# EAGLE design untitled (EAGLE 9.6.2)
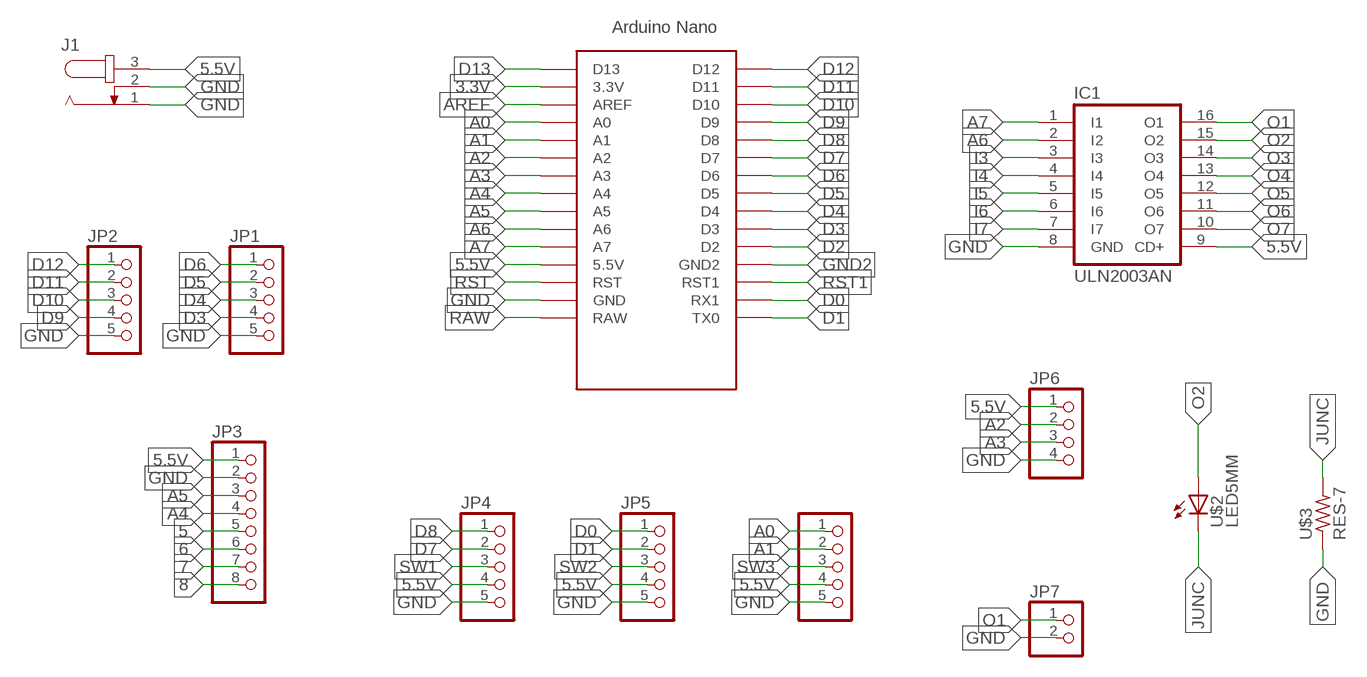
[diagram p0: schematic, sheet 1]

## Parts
3_ENCODERS  PINHD-1X5  [1X05]
IC1  ULN2003AN  [DIL16]
J1  JACK-PLUG0  [SPC4077]
JP1  PINHD-1X5  [1X05]
JP2  PINHD-1X5  [1X05]
JP3  PINHD-1X8  [1X08]
JP4  PINHD-1X5  [1X05]
JP5  PINHD-1X5  [1X05]
JP6  PINHD-1X4  [1X04]
JP7  PINHD-1X2  [1X02]
U$1  ARDUINO_NANO  [NANO]
U$2  LED5MM  [LED5MM]
U$3  RES-7  [0204/7]

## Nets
3.3V: U$1.3.3V
5: JP3.5
5.5V: 3_ENCODERS.4 IC1.9(CD+) J1.3 JP3.1 JP4.4 JP5.4 JP6.1 U$1.5V(5.5V)
6: JP3.6
7: JP3.7
8: JP3.8
A0: 3_ENCODERS.1 U$1.A0
A1: 3_ENCODERS.2 U$1.A1
A2: JP6.2 U$1.A2
A3: JP6.3 U$1.A3
A4: JP3.4 U$1.A4
A5: JP3.3 U$1.A5
A6: IC1.2(I2) U$1.A6
A7: IC1.1(I1) U$1.A7
AREF: U$1.AREF
D0: JP5.1 U$1.RX1
D1: JP5.2 U$1.TX0
D2: U$1.D2
D3: JP1.4 U$1.D3
D4: JP1.3 U$1.D4
D5: JP1.2 U$1.D5
D6: JP1.1 U$1.D6
D7: JP4.2 U$1.D7
D8: JP4.1 U$1.D8
D9: JP2.4 U$1.D9
D10: JP2.3 U$1.D10
D11: JP2.2 U$1.D11
D12: JP2.1 U$1.D12
D13: U$1.D13
GND: 3_ENCODERS.5 IC1.8(GND) J1.1 J1.2 JP1.5 JP2.5 JP3.2 JP4.5 JP5.5 JP6.4 JP7.2 U$1.GND U$3.1
GND2: U$1.GND1(GND2)
I3: IC1.3(I3)
I4: IC1.4(I4)
I5: IC1.5(I5)
I6: IC1.6(I6)
I7: IC1.7(I7)
JUNC: U$2.K(C) U$3.2
O1: IC1.16(O1) JP7.1
O2: IC1.15(O2) U$2.A
O3: IC1.14(O3)
O4: IC1.13(O4)
O5: IC1.12(O5)
O6: IC1.11(O6)
O7: IC1.10(O7)
RAW: U$1.RAW
RST: U$1.RST
RST1: U$1.RST1
SW1: JP4.3
SW2: JP5.3
SW3: 3_ENCODERS.3

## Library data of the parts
3_ENCODERS JP1 JP2 JP4 JP5 = MIA-Training:PINHD-1X5: PIN HEADER
IC1 = MIA-Training:ULN2003A: DRIVER ARRAY
J1 = con-jack:JACK-PLUG: DC POWER JACK Power Jack, DC, Right Angle, Through Hole, Rated 5A at 16VDC, PC Terminals Distributor: Farnell (www.Farnell.de) Drawing: 84N1161.pdf / 84N1162.pdf Manufacturer: SPC Technology (www.spctechnology.com) Type: SPC4077 / SPC 4078; OC_FARNELL: unknown; OC_NEWARK: unknown
JP3 = MIA-Training:PINHD-1X8: PIN HEADER
JP6 = MIA-Training:PINHD-1X4: PIN HEADER
JP7 = MIA-Training:PINHD-1X2: PIN HEADER
U$1 = MIA-Training:ARDUINO_NANO: Arduino Nano
U$2 = MIA-Training:LED5MM
U$3 = MIA-Training:RES-7

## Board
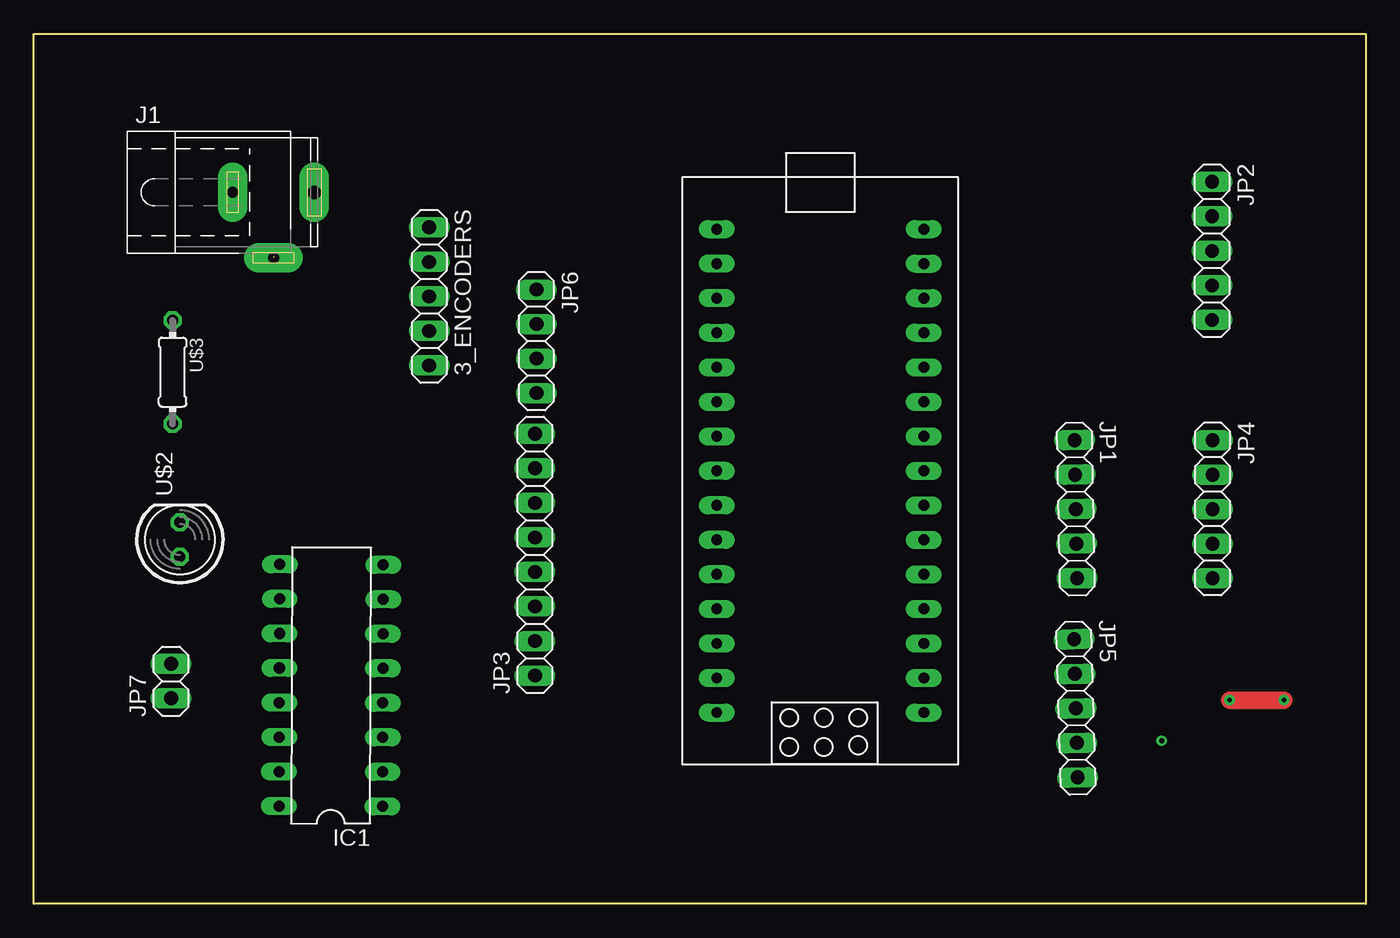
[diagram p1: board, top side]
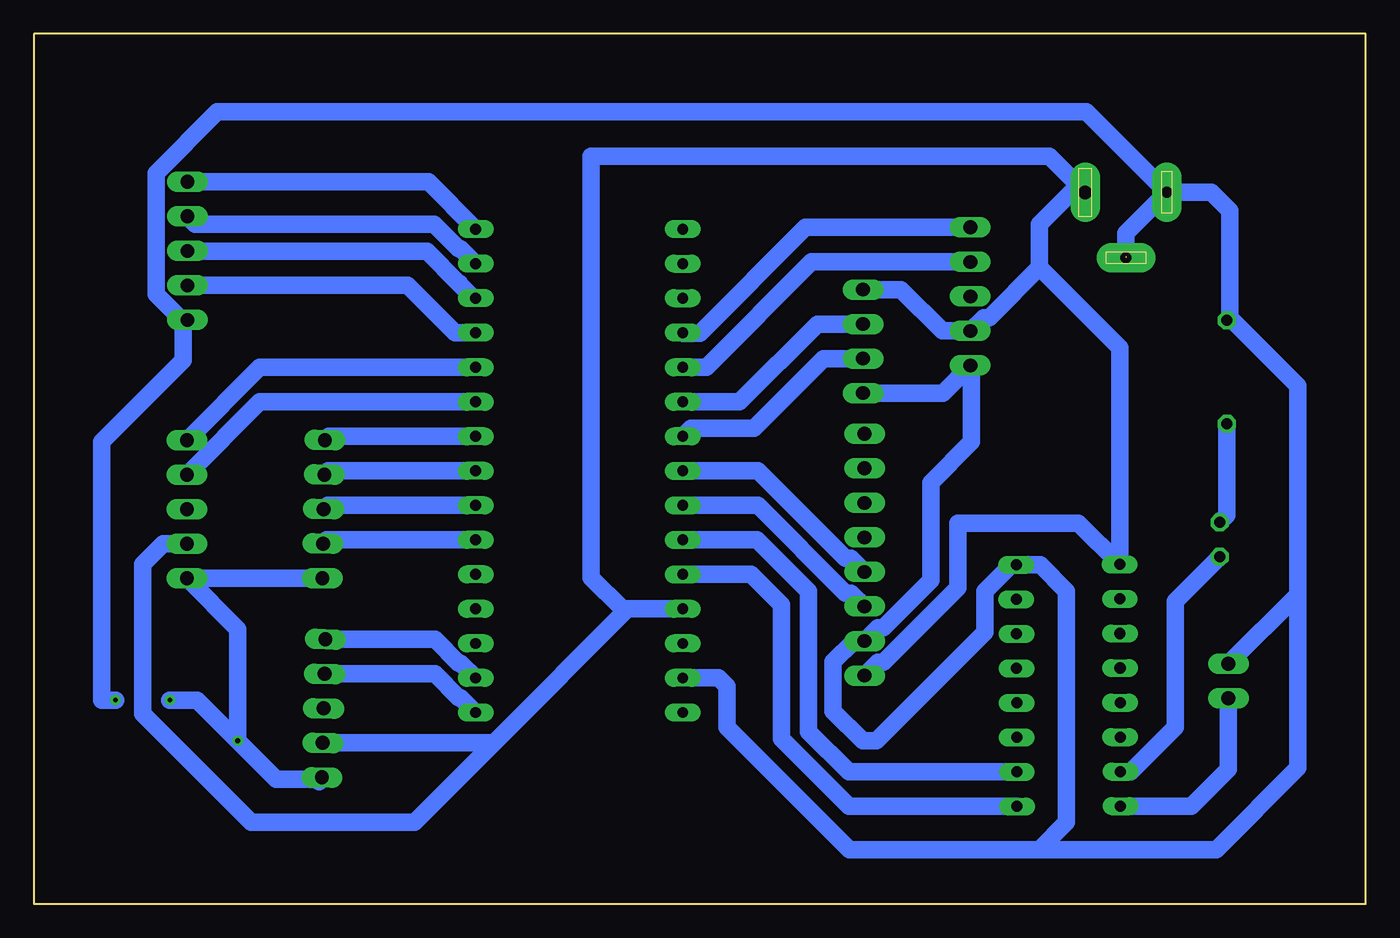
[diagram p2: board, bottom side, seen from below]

Size 98 x 64 mm. Coordinates in mm from the lower left corner, seen from the top.
Outline: 0,0 0,64 98,64 98,0 0,0
Copper layers (1*16): Top 0.035mm / dielectric 1.5mm / Bottom 0.035mm
Design rules "default": minimum track width 6mil, minimum drill 0.35mm, track to track 6mil, track to pad 6mil, pad to pad 6mil, via to via 6mil, smd to smd 6mil, copper to edge 40mil, drill to drill 6mil, minimum pad ring 10mil, minimum via ring 8mil, stop-mask expansion 4mil, vias tented up to drill 0mil, thermal gap 10mil

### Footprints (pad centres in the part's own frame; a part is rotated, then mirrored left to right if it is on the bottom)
1X05 = drill 1.016 long: 1 -5.08,0; 2 -2.54,0; 3 0,0; 4 2.54,0; 5 5.08,0
DIL16 = drill 0.813 long: 1 -8.89,-3.81; 2 -6.35,-3.81; 3 -3.81,-3.81; 4 -1.27,-3.81; 5 1.27,-3.81; 6 3.81,-3.81; 7 6.35,-3.81; 8 8.89,-3.81; 9 8.89,3.81; 10 6.35,3.81; 11 3.81,3.81; 12 1.27,3.81; 13 -1.27,3.81; 14 -3.81,3.81; 15 -6.35,3.81; 16 -8.89,3.81
SPC4077 = drill 0.8 pad 2.184 long: 1 -3,0; 2 0,-4.8 | drill 1 pad 2.184 long: 3 3,0
1X08 = drill 1.016 long: 1 -8.89,0; 2 -6.35,0; 3 -3.81,0; 4 -1.27,0; 5 1.27,0; 6 3.81,0; 7 6.35,0; 8 8.89,0
1X04 = drill 1.016 long: 1 -3.81,0; 2 -1.27,0; 3 1.27,0; 4 3.81,0
1X02 = drill 1.016 long: 1 -1.27,0; 2 1.27,0
NANO = drill 0.8 long: 3.3V -10.16,24.13; 5V -10.16,-1.27; A0 -10.16,19.05; A1 -10.16,16.51; A2 -10.16,13.97; A3 -10.16,11.43; A4 -10.16,8.89; A5 -10.16,6.35; A6 -10.16,3.81; A7 -10.16,1.27; AREF -10.16,21.59; D2 5.08,1.27; D3 5.08,3.81; D4 5.08,6.35; D5 5.08,8.89; D6 5.08,11.43; D7 5.08,13.97; D8 5.08,16.51; D9 5.08,19.05; D10 5.08,21.59; D11 5.08,24.13; D12 5.08,26.67; D13 -10.16,26.67; GND -10.16,-6.35; GND1 5.08,-1.27; RAW -10.16,-8.89; RST -10.16,-3.81; RST1 5.08,-3.81; RX1 5.08,-6.35; TX0 5.08,-8.89
LED5MM = drill 0.813 octagon: A -1.27,0; K 1.27,0
0204/7 = drill 0.813 octagon: 1 -3.81,0; 2 3.81,0

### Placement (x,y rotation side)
3_ENCODERS  29.09,44.69 270 top
IC1  21.87,16.07 89.8 top
J1  17.63,52.35 0 top
JP1  76.68,29.04 271.1 top
JP2  86.71,48.04 270 top
JP3  36.87,25.69 90 top
JP4  86.74,29.04 270 top
JP5  76.68,14.39 271.5 top
JP6  36.98,41.39 270 top
JP7  10.09,16.39 90 top
U$1  60.41,22.97 0 top
U$2  10.74,26.8 90 top
U$3  10.2,39.12 270 top

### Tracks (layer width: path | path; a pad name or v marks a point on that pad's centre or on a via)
5.5V
  Bottom 1.27: 24,46.83 27.69,43.14 28.1,43.14 3_ENCODERS.4 31.15,42.15 34.2,45.2 JP6.1 | JP3.1 35.88,17.79 35.47,17.79 30,23.26 30,28 21.12,28 IC1.9 18.09,40.92 24,46.83 | 64.15,11.85 JP5.4 75.85,11.85 | 64.15,11.85 64,12 54.3,21.7 U$1.5V 54.7,21.7 57,24 57,55 23.28,55 J1.3 21.65,52.35 24,50 24,46.83 | JP4.4 88.5,26.5 90,25 90,14 82,6 70,6 64.15,11.85
A0
  Bottom 1.27: 3_ENCODERS.1 41.23,49.77 49,42 50.23,42 U$1.A0
A1
  Bottom 1.27: 3_ENCODERS.2 40.77,47.23 48.52,39.48 U$1.A1
A2
  Bottom 1.27: JP6.2 40.34,42.66 46.06,36.94 U$1.A2
A3
  Bottom 1.27: JP6.3 39.88,40.12 45,35 49.65,35 U$1.A3
A4
  Bottom 1.27: JP3.4 37.86,25.41 38.27,25.41 44.72,31.86 U$1.A4
A5
  Bottom 1.27: JP3.3 37.86,22.87 38.27,22.87 44.72,29.32 U$1.A5
A6
  Bottom 1.27: IC1.2 38.02,9.71 41,12.68 41,23 44.78,26.78 U$1.A6
A7
  Bottom 1.27: IC1.1 38.02,7.17 43,12.14 43,22 45.24,24.24 U$1.A7
D0
  Bottom 1.27: U$1.RX1 66.59,17.72 66.74,17.72 68.49,19.47 JP5.1
D1
  Bottom 1.27: U$1.TX0 66.59,15.18 66.74,15.18 68.49,16.93 JP5.2
D3
  Bottom 1.27: JP1.4 76.45,26.78 U$1.D3
D4
  Bottom 1.27: JP1.3 76.4,29.32 73,29.32 | 73,29.32 U$1.D4 | 73,29.32
D5
  Bottom 1.27: JP1.2 76.35,31.86 U$1.D5
D6
  Bottom 1.27: JP1.1 76.3,34.4 U$1.D6
D7
  Bottom 1.27: U$1.D7 81.38,36.94 JP4.2
D8
  Bottom 1.27: U$1.D8 81.38,39.48 JP4.1
D9
  Bottom 1.27: JP2.4 70.5,45.5 67.02,42.02 U$1.D9
D10
  Bottom 1.27: JP2.3 86.67,48 69.08,48 66.74,45.66 | 66.74,45.66 66.66,45.66 | 66.74,45.66 65.64,44.56 U$1.D10
D11
  Bottom 1.27: JP2.2 86.13,50 68.54,50 66.74,48.2 66.59,48.2 U$1.D11
D12
  Bottom 1.27: JP2.1 68.97,53.12 U$1.D12
GND  (via drill 0.35)  (1 unrouted)
  Top 1.27: v92,15 v88,15
  Bottom 1.27: J1.1 11.35,52.35 10,51 10,43.13 | 10,43.13 U$3.1 | JP6.4 31.12,37.58 3_ENCODERS.5 29,39.52 29,34 32,31 32,23.8 35.47,20.33 35.88,20.33 JP3.2 37.66,19.34 39.18,17.82 39.18,14.18 37,12 36,12 28,20 28,23 26.05,24.95 IC1.8 23.95,24.95 22,23 22,6 24,4 | JP7.2 5,22.75 | 10,43.13 5,38.13 5,22.75 | J1.1 20.55,58.27 84.51,58.27 89.02,53.76 89.02,44.86 87.12,42.96 JP2.5 87,42.67 87,40 93,34 93,15 v92,15 | JP4.5 JP1.5 | 24,4 38,4 47,13 47,16 47.62,16.62 U$1.GND | 87.15,23.96 JP4.5 | 24,4 11,4 5,10 5,22.75 | J1.1 17.63,49.35 17.63,47.63 | 77,9 76.81,9.19 | 76.81,9.19 JP5.5 | JP4.5 83,20.22 v83,12 | 76.81,9.19 80.19,9.19 v83,12 | v88,15 86,15 v83,12
JUNC
  Bottom 1.27: U$3.2 10.2,28.61 U$2.K
O1
  Bottom 1.27: IC1.16 12.81,7.19 10.09,9.91 JP7.1
O2
  Bottom 1.27: U$2.A 14,22.27 14,13 17.27,9.73 IC1.15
